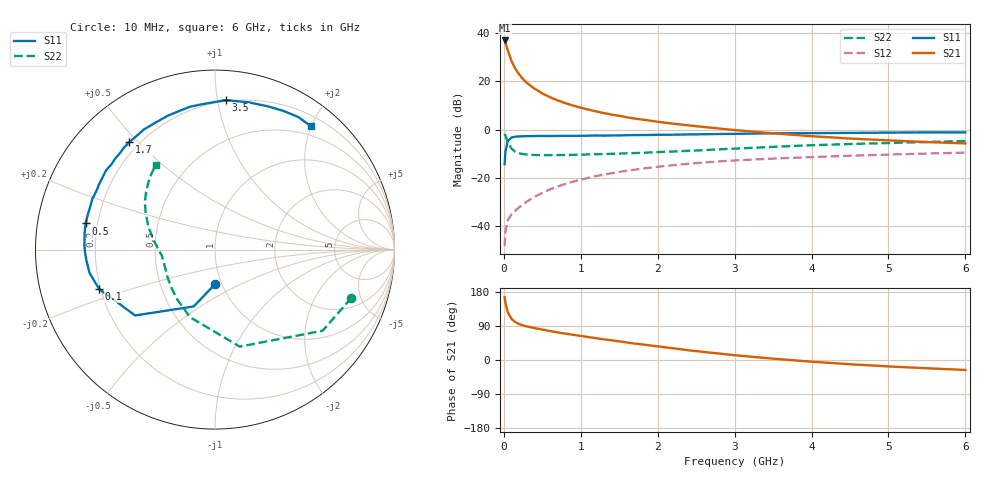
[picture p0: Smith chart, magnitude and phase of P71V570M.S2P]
! SIEMENS Small Signal Semiconductors
! BFP196
! Si NPN RF Bipolar Junction Transistor in SOT143
! VCE = 1.5 V  IC = 70 mA
! Common Emitter S-Parameters:  May  1996
# GHz  S  MA  R  50
!  f  S11  S21  S12  S22
! GHz  MAG  ANG  MAG  ANG  MAG  ANG  MAG  ANG
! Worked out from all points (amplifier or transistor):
!   36 points, 10 MHz to 6 GHz, reference 50 ohm
!   highest |S21| = 37.0 dB at 10 MHz (marker M1)
!   |S21| within 3 dB of that: start of sweep to 40.83 MHz
!   unconditionally stable (mu >= 1): 321.6 MHz to 5.243 GHz; 5.783 GHz to end of sweep
!   at 250 MHz: K = 0.94, MSG = 26.0 dB, |S12| = -31.0 dB
!   at 1.4 GHz: K = 1.11, MAG = 10.2 dB, |S12| = -18.2 dB
!   at 6 GHz: K = 1.01, MAG = 1.5 dB, |S12| = -9.6 dB
!   S11 on the Smith chart (normalised r, x): 10 MHz: 0.93, -0.37; 100 MHz: 0.19, -0.16; 500 MHz: 0.15, +0.10; 1.7 GHz: 0.16, +0.47; 3.5 GHz: 0.19, +1.06; 6 GHz: 0.35, +1.99
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0.01  0.1909 -89.5  70.44 165.5  0.0038 77.1  0.8065 -19.5
0.02  0.3381 -110.5  64.13 151.9  0.0075 65.1  0.7508 -37.0
0.05  0.5767 -140.5  44.64 126.6  0.0131 52.6  0.5579 -75.7
0.1  0.6817 -161.2  26.25 108.4  0.0174 50.8  0.4012 -110.3
0.15  0.7111 -169.5  18.19 100.0  0.0208 52.5  0.346 -128.4
0.2  0.719 -175.3  13.84 94.8  0.0244 56.2  0.3211 -139.5
0.25  0.7249 -179.0  11.07 91.2  0.0281 58.7  0.309 -147.3
0.3  0.7281 178.2  9.283 88.6  0.0321 61.0  0.3029 -152.2
0.4  0.7324 172.6  7.015 84.1  0.0403 63.7  0.2962 -159.4
0.5  0.736 168.6  5.617 80.3  0.0487 65.1  0.2946 -164.0
0.6  0.7349 164.5  4.683 76.4  0.0572 64.9  0.2944 -167.1
0.7  0.7357 160.7  4.024 72.7  0.0657 64.9  0.2956 -169.5
0.9  0.7369 153.8  3.141 66.5  0.083 63.4  0.2982 -173.3
1.1  0.745 147.1  2.586 60.4  0.0996 61.3  0.3044 -176.1
1.3  0.7476 140.6  2.195 54.6  0.1162 58.3  0.31 -178.8
1.7  0.7657 128.5  1.687 43.3  0.1469 52.7  0.3248 176.3
2.2  0.781 115.1  1.322 30.9  0.1821 44.8  0.3492 170.4
2.8  0.808 99.9  1.048 17.0  0.2179 35.7  0.3889 161.8
3.5  0.8351 85.9  0.832 3.5  0.2497 25.4  0.4368 152.2
4.5  0.8511 69.7  0.65 -11.2  0.2859 13.3  0.5003 140.1
5.5  0.8725 57.8  0.548 -21.8  0.3174 2.4  0.5516 130.0
6  0.8706 52.2  0.516 -26.3  0.3316 -3.3  0.575 125.0
